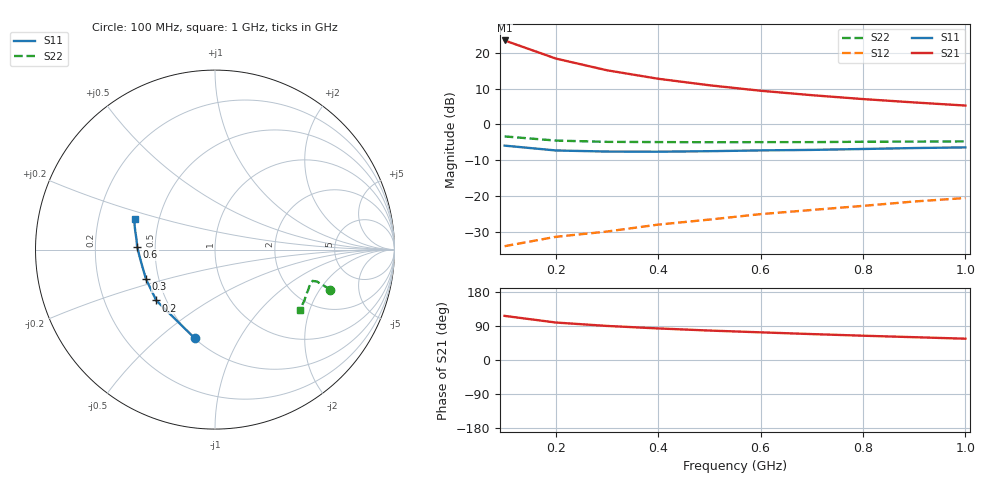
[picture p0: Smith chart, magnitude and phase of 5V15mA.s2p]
#  HZ  S  MA  R  50.0000
! Device:15GN03CA
! "! Bias:VCE=5V, IC=15mA  "
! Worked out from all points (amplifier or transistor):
!   10 points, 100 MHz to 1 GHz, reference 50 ohm
!   highest |S21| = 23.4 dB at 100 MHz (marker M1)
!   |S21| within 3 dB of that: start of sweep to 159.4 MHz
!   unconditionally stable (mu >= 1): 175.8 MHz to end of sweep
!   at 200 MHz: K = 1.12, MAG = 22.8 dB, |S12| = -31.4 dB
!   at 600 MHz: K = 1.51, MAG = 13.0 dB, |S12| = -25.0 dB
!   at 1 GHz: K = 1.31, MAG = 9.6 dB, |S12| = -20.5 dB
!   S11 on the Smith chart (normalised r, x): 100 MHz: 0.50, -0.66; 200 MHz: 0.44, -0.31; 300 MHz: 0.42, -0.17; 600 MHz: 0.39, +0.02; 1 GHz: 0.36, +0.16
1e8  0.506 -103.0  14.84 116.4  0.02 52.2  0.68 -19.1
2e8  0.433 -139.1  8.3 98.9  0.027 55.3  0.595 -17.4
3e8  0.418 -156.7  5.691 89.9  0.032 60.5  0.571 -17.8
4e8  0.416 -167.5  4.336 83.3  0.04 65.0  0.567 -19.2
5e8  0.423 -175.6  3.518 77.7  0.047 70.8  0.564 -21.4
6e8  0.434 177.9  2.949 73.0  0.056 75.4  0.566 -23.8
7e8  0.441 172.6  2.558 68.4  0.064 77.2  0.566 -26.4
8e8  0.454 167.7  2.257 64.1  0.073 80.3  0.573 -29.4
9e8  0.468 163.2  2.026 60.2  0.084 82.2  0.576 -32.6
1e9  0.478 159.4  1.833 56.2  0.094 82.8  0.579 -35.4
